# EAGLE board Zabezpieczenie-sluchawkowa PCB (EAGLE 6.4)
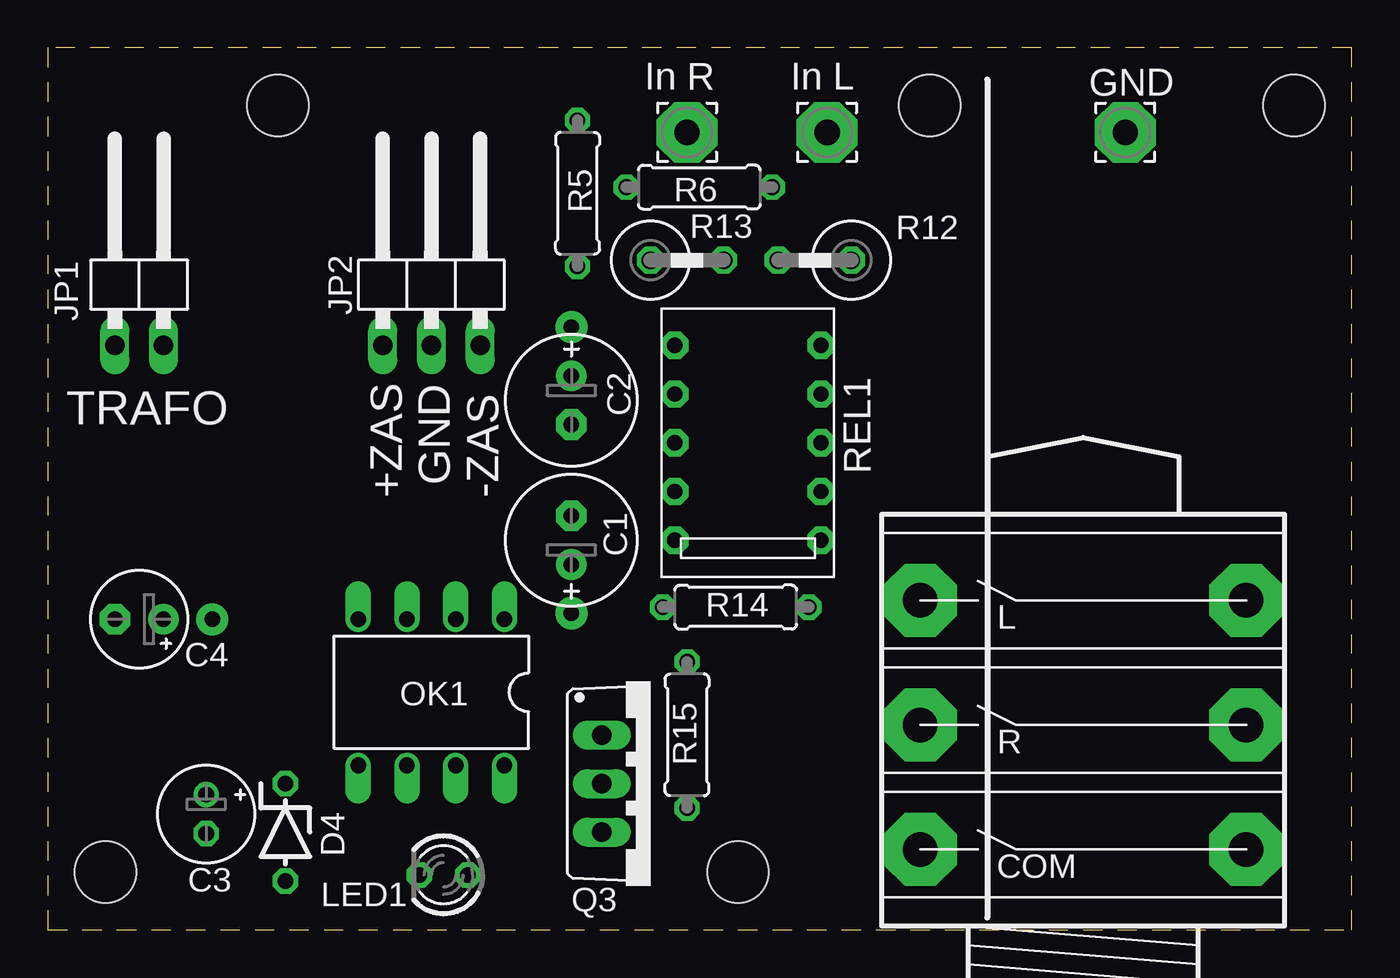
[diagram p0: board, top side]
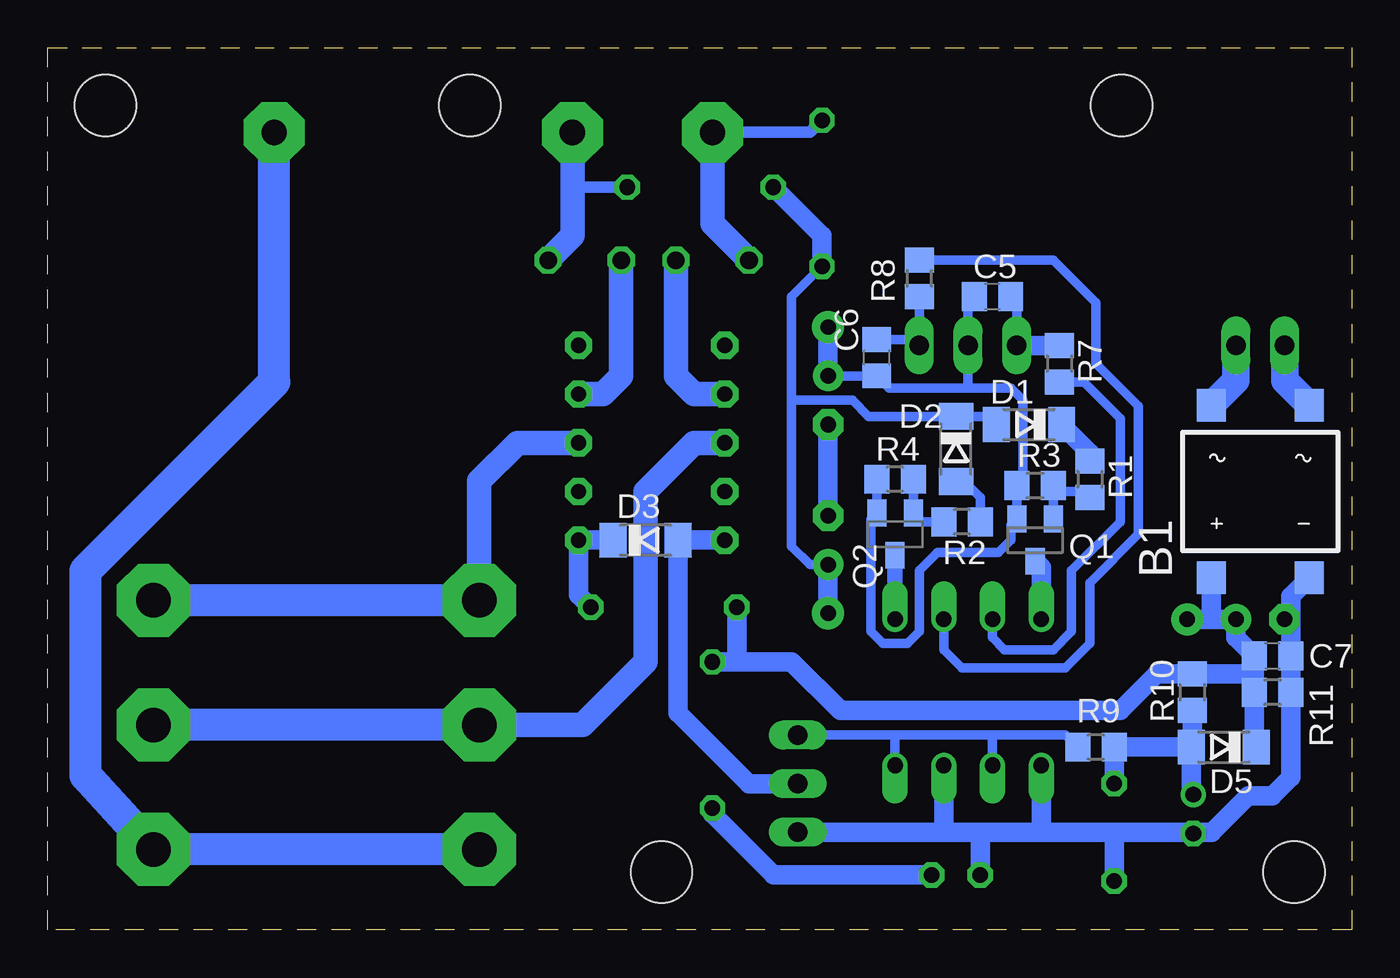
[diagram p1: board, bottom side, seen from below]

Size 68 x 46 mm. Coordinates in mm from the lower left corner, seen from the top.
Outline: 0,0 68,0 68,46 0,46 0,0
Copper layers (1*16): Top 0.035mm / dielectric 1.5mm / Bottom 0.035mm
Design rules "AVT-Elmax": minimum track width 8mil, minimum drill 18mil, track to track 8mil, track to pad 8mil, pad to pad 8mil, via to via 8mil, smd to smd 8mil, copper to edge 10mil, drill to drill 8mil, minimum pad ring 10mil, minimum via ring 8mil, stop-mask expansion 4mil, vias tented up to drill 0mil, thermal gap 10mil
Holes 3.2 mm at 3,3 36,3 46,43 12,43 65,43

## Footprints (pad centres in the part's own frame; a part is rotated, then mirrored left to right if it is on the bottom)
DFS = smd 1.5 x 1.7: + -2.55,-4.5; - 2.55,-4.5; AC1 -2.55,4.5; AC2 2.55,4.5
E2,5-7 = drill 0.813 pad 1.6: + -1.27,0 | drill 0.813 pad 1.6 octagon: - 1.27,0
E2-5 = drill 0.813 pad 1.27: + -1.016,0 | drill 0.813 pad 1.27 octagon: - 1.016,0
E2,5-5 = drill 0.813 pad 1.6: + -1.27,0 | drill 0.813 pad 1.6 octagon: - 1.27,0
C0805 = smd 1.3 x 1.5: 1 -0.95,0; 2 0.95,0
JACK6.3-6PIN = drill 1.8 pad 3.81 octagon: P$1 2,17.5; P$2 2,11; P$3 2,4.5; P$4 19,4.5; P$5 19,11; P$6 19,17.5
SOD80C = smd 1.4 x 1.8: A 1.7,0; C -1.7,0
ZDIO-5 = drill 0.813 octagon: A 2.54,0; C -2.54,0
1X02/90 = drill 1.016 long: 1 -1.27,-3.81; 2 1.27,-3.81
1X03/90 = drill 1.016 long: 1 -2.54,-3.81; 2 0,-3.81; 3 2.54,-3.81
LED3MM = drill 0.813 octagon: A -1.27,0; K 1.27,0
DIL08 = drill 0.813 offset: 1 -3.81,-3.81; 2 -1.27,-3.81; 3 1.27,-3.81; 4 3.81,-3.81; 5 3.81,3.81; 6 1.27,3.81; 7 -1.27,3.81; 8 -3.81,3.81
3,17/1,3 = drill 1.321 pad 3.175 octagon: 1 0,0
SOT23 = smd 1 x 1.4: 1 -0.95,-1.1; 2 0.95,-1.1; 3 0,1.1
SOT23-BEC = smd 1 x 1.4: B -0.95,-1.1; C 0,1.1; E 0.95,-1.1
TO220BV = drill 1.016 long: D 0,-2.54; G -2.54,-2.54; S 2.54,-2.54
R0805 = smd 1.3 x 1.5: 1 -0.95,0; 2 0.95,0
0207/7 = drill 0.813 octagon: 1 -3.81,0; 2 3.81,0
0411V = drill 0.914 octagon: 1 -2.54,0; 2 1.27,0
AZ850 = drill 0.8 pad 1.422 octagon: + -5.08,-3.81; - -5.08,3.81; COM1 0,3.81; COM2 0,-3.81; NC1 -2.54,3.81; NC2 -2.54,-3.81; NO1 2.54,3.81; NO2 2.54,-3.81; P$5 5.08,-3.81; P$6 5.08,3.81

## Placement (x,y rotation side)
B1  DF06S  [DFS]  4.76,22.86 0 bottom
C1  47u T  [E2,5-7]  27.3,20.32 90 top
C2  47u T  [E2,5-7]  27.3,27.62 270 top
C3  10u  [E2-5]  8.26,6.03 270 top
C4  47u  [E2,5-5]  4.76,16.19 180 top
C5  100n  [C0805]  18.73,33.02 180 bottom
C6  100n  [C0805]  24.77,29.84 90 bottom
C7  100n  [C0805]  4.13,14.29 0 bottom
CON1  JACK6.3-6PIN  [JACK6.3-6PIN]  43.5,-0.32 0 top
D1  1N4148  [SOD80C]  16.83,26.35 180 bottom
D2  1N4148  [SOD80C]  20.64,25.08 270 bottom
D3  1N4148  [SOD80C]  36.83,20.32 0 bottom
D4  15V  [ZDIO-5]  12.38,5.08 270 top
D5  1N4148  [SOD80C]  6.67,9.53 180 bottom
JP1  Trafo  [1X02/90]  4.76,34.29 0 top
JP2  Zasilanie  [1X03/90]  20,34.29 0 top
LED1  [LED3MM]  20.64,2.86 180 top
OK1  LTV826  [DIL08]  20,12.38 180 top
PAD1  In R  [3,17/1,3]  33.34,41.59 0 top
PAD2  In L  [3,17/1,3]  40.64,41.59 0 top
PAD3  COM  [3,17/1,3]  56.2,41.59 0 top
Q1  BC846  [SOT23]  16.51,20.32 180 bottom
Q2  BC858  [SOT23-BEC]  23.81,20.64 180 bottom
Q3  IRF520  [TO220BV]  31.43,7.62 270 top
R1  33k  [R0805]  13.65,23.5 270 bottom
R2  33k  [R0805]  20.32,21.27 180 bottom
R3  *  [R0805]  16.51,23.18 0 bottom
R4  *  [R0805]  23.81,23.5 180 bottom
R5  22k  [0207/7]  27.62,38.42 270 top
R6  22k  [0207/7]  33.97,38.73 180 top
R7  4k7  [R0805]  15.24,29.53 270 bottom
R8  4k7  [R0805]  22.54,33.97 90 bottom
R9  4k7  [R0805]  13.34,9.53 180 bottom
R10  1M  [R0805]  8.3,12.38 90 bottom
R11  *  [R0805]  4.13,12.38 180 bottom
R12  *  [0411V]  39.37,34.92 180 top
R13  *  [0411V]  33.97,34.92 0 top
R14  *  [0207/7]  35.88,16.83 0 top
R15  RLED  [0207/7]  33.34,10.16 90 top
REL1  AZ850  [AZ850]  36.51,25.4 90 top

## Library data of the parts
B1 = rectifier
C1-C7 R1-R15 = rcl
CON1 = con-jack2
D1-D5 = diode
JP1 JP2 = pinhead
LED1 = led
OK1 = optocoupler; OC_FARNELL: unknown; OC_NEWARK: unknown
PAD1-PAD3 = wirepad
Q1 = transistor-npn
Q2 = transistor-pnp
Q3 = transistor-power
REL1 = relay

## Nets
GND: C2.+ C5.2 C6.1 JP2.2 Q1.2 Q2.E R3.1 R4.2
N$1: D1.C R1.1
N$2: Q1.1 R1.2 R3.2
N$3: Q2.B R2.2 R4.1
N$4: OK1.2 R8.2
N$5: D2.A R2.1
N$6: D3.A Q3.D REL1.-
N$7: C1.- C2.-
N$8: OK1.1 Q2.C
N$9: OK1.3 R7.2
N$10: OK1.4 Q1.3
N$11: PAD2.1 R6.1 R12.1
N$12: B1.+ C4.+ C7.1 D5.C R10.2 R11.2 R14.1 R15.2
N$13: OK1.6 OK1.8 Q3.G R9.2
N$14: B1.- C3.- C4.- C7.2 D4.A LED1.K OK1.5 OK1.7 Q3.S R11.1
N$15: C3.+ D4.C D5.A R9.1 R10.1
N$16: C1.+ D1.A D2.C R5.2 R6.2
N$17: PAD1.1 R5.1 R13.1
N$18: B1.AC2 JP1.1
N$19: B1.AC1 JP1.2
N$20: R13.2 REL1.NO1
N$21: R12.2 REL1.NO2
N$22: CON1.P$3 CON1.P$4 PAD3.1
N$23: CON1.P$1 CON1.P$6 REL1.COM2
N$24: CON1.P$2 CON1.P$5 REL1.COM1
N$25: D3.C R14.2 REL1.+
N$26: LED1.A R15.1
VCC: C5.1 JP2.1 R7.1
VSS: C6.2 JP2.3 R8.1

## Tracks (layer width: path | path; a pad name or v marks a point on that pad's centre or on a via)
GND  (via drill 0.8 pad 1.68)
  Bottom 0.508: Q2.E R4.2 | Q2.E 24.76,21.59 | Q2.E 25.08,21.42 25.08,15.56 24.45,14.92 23.18,14.92 22.54,15.56 22.54,18.73 21.59,19.68 18.41,19.68 17.78,20.32 17.78,21.1 Q1.2 R3.1 17.14,23.49 17.14,27.62 17.78,28.26 20,28.26 | 20,28.26 JP2.2 20,32.7 C5.2 | C2.+ C6.1 24.13,28.26 20,28.26
  Bottom 1.016: v27.3,31.43 C2.+
N$1
  Bottom 1.016: R1.1 13.65,24.88 D1.C
N$2
  Bottom 0.508: 15.56,21.91 Q1.1 | 15.56,21.91 R3.2 15.24,22.86 13.97,22.86 R1.2 | 15.56,21.91
N$3
  Bottom 0.508: R4.1 Q2.B 22.4,21.27 R2.2
N$4
  Bottom 0.508: OK1.2 21.27,14.61 20.32,13.65 14.92,13.65 13.65,14.92 13.65,18.1 11.11,20.64 11.11,27.3 13.34,29.53 13.34,32.7 15.55,34.92 R8.2
N$5
  Bottom 0.508: R2.1 19.37,22.55 20.21,23.38 D2.A
N$6
  Bottom 1.016: REL1.- D3.A 35.13,11.32 31.43,7.62 Q3.D
N$7
  Bottom 1.016: C1.- C2.-
N$8
  Bottom 0.813: OK1.1 Q2.C
N$9
  Bottom 0.508: OK1.3 18.73,15.24 18.1,14.61 15.56,14.61 14.61,15.56 14.61,18.73 12.06,21.27 12.06,26.67 13.97,28.57 R7.2
N$10
  Bottom 1.016: Q1.3 16.19,18.9 OK1.4
N$11
  Bottom 0.61: 40.64,38.73 R6.1
  Bottom 1.27: PAD2.1 40.64,38.73 40.64,36.2 R12.1
N$12  (via drill 0.8 pad 1.68)
  Bottom 1.016: R11.2 C7.1 6.03,15.24 C4.+ 7.3,16.19 | R11.2 5.08,13.33 R10.2 10.16,13.33 12.06,11.43 26.67,11.43 29.21,13.97 32.07,13.97 | R11.2 5.08,9.63 D5.C | 32.07,13.97 R15.2 | 32.07,13.97 R14.1 | 7.3,16.19 v8.57,16.19 | B1.+ 7.31,16.2 7.3,16.19
N$13
  Bottom 0.508: 18.73,10.16 OK1.6 | 18.73,10.16 14.92,10.16 R9.2 | 18.73,10.16 23.81,10.16 | 23.81,10.16 Q3.G | 23.81,10.16 OK1.8
N$14
  Bottom 1.016: 8.26,5.08 7.3,5.08 5.4,6.99 4.13,6.99 3.18,7.93 R11.1 C7.2 3.18,16.51 | 8.26,5.08 C3.- | 8.26,5.08 12.38,5.08 | 12.38,5.08 16.19,5.08 | 16.19,5.08 19.37,5.08 | 19.37,5.08 21.27,5.08 | 21.27,5.08 Q3.S | 21.27,5.08 OK1.7 | 16.19,5.08 OK1.5 | 12.38,5.08 D4.A | 19.37,5.08 LED1.K | 3.18,16.51 3.18,17.39 B1.- | C4.- 3.18,16.51
N$15
  Bottom 1.016: D4.C R9.1 D5.A | D5.A 8.37,7.48 C3.+ | R10.1 8.3,9.59 D5.A
N$16  (via drill 0.8 pad 1.68)
  Bottom 0.508: C1.+ 28.26,19.05 29.21,20 29.21,27.62 | 29.21,27.62 29.21,33.02 R5.2 | 29.21,27.62 26.04,27.62 25.2,26.78 D2.C 18.96,26.78 D1.A
  Bottom 1.016: R5.2 27.62,36.2 R6.2 | v27.3,16.51 C1.+
N$17
  Bottom 0.61: PAD1.1 28.26,41.59 R5.1
  Bottom 1.27: PAD1.1 33.34,36.83 R13.1
N$18
  Bottom 1.422: JP1.1 3.49,28.64 B1.AC2
N$19
  Bottom 1.422: JP1.2 6.03,28.64 B1.AC1
N$20
  Bottom 1.27: REL1.NO1 34.29,27.94 35.24,28.89 R13.2
N$21
  Bottom 1.27: REL1.NO2 39.05,27.94 38.1,28.89 R12.2
N$22
  Bottom 1.676: CON1.P$3 CON1.P$4 66.04,8.04 66.04,18.73 56.2,28.57 PAD3.1
N$23
  Bottom 1.27: REL1.COM2 43.5,25.4 45.5,23.4 CON1.P$1
  Bottom 1.676: CON1.P$1 CON1.P$6
N$24
  Bottom 1.27: REL1.COM1 34.29,25.4 36.83,22.86 36.83,13.97 40.12,10.68 CON1.P$2
  Bottom 1.676: CON1.P$2 CON1.P$5
N$25
  Bottom 1.016: D3.C REL1.+ 40.32,17.46 R14.2
N$26
  Bottom 1.016: LED1.A 30.16,2.86 33.34,6.03 R15.1
VCC
  Bottom 0.508: JP2.1 17.46,32.7 C5.1
  Bottom 1.016: R7.1 JP2.1
VSS
  Bottom 0.508: R8.1 JP2.3 22.54,30.8 C6.2

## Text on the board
tPlace: In R | In L | GND | TRAFO | +ZAS / GND / -ZAS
